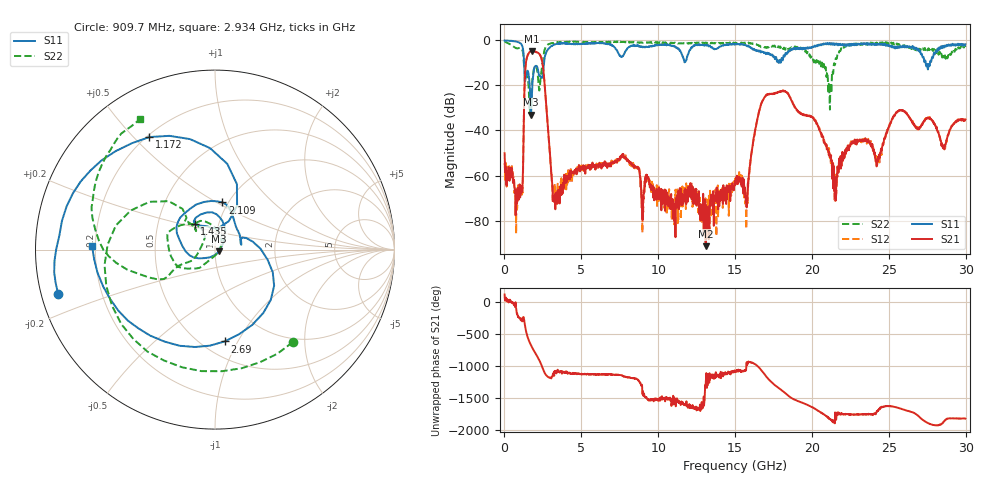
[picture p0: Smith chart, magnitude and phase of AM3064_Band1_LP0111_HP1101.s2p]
# Hz S DB R 50.0
!freq dBS11 angS11 dBS21 angS21 dBS12 angS12 dBS22 angS22
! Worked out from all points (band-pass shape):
!   1600 points, 10 MHz to 29.98 GHz, reference 50 ohm
!   highest |S21| = -4.65 dB at 1.791 GHz (marker M1); lowest = -91.4 dB at 13.09 GHz (marker M2)
!   |S21| within 3 dB of the highest: 1.46 GHz to 2.392 GHz (932.2 MHz wide, 48.4 % of centre)
!   lowest |S11| = -32.9 dB at 1.716 GHz (marker M3), VSWR 1.05, Z = 52.1 - j0.908 ohm
!   |S11| at or under -10 dB: 1.277 GHz to 2.567 GHz (1.29 GHz wide, 67.1 % of centre); 17.8465 GHz to 17.85471 GHz (8.204 MHz wide, 0.046 % of centre); 27.4 GHz to 27.68 GHz (283.1 MHz wide, 1.03 % of centre)
!   |S22| runs from -32.7 to -0.3 dB; largest |S21 - S12| = 0.009
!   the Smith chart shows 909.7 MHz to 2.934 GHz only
!   S11 on the Smith chart (normalised r, x): 909.7 MHz: 0.05, -0.14; 1.172 GHz: 0.21, +0.56; 1.435 GHz: 0.77, +0.23; 2.109 GHz: 0.94, +0.53; 2.69 GHz: 0.64, -0.88; 2.934 GHz: 0.19, +0.02
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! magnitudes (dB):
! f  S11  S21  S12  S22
! 10 MHz  0.0  -50.1  -54.5  -0.3
! 909.7 MHz  -0.8  -66.5  -63.4  -3.4
! 1.172 GHz  -2.8  -65.2  -67.7  -4.5
! 1.435 GHz  -14.8  -8.4  -8.3  -15.9
! 1.716 GHz  -32.9  -4.7  -4.7  -25.5
! 1.791 GHz  -22.5  -4.6  -4.6  -18.6
! 2.109 GHz  -11.5  -5.3  -5.3  -12.7
! 2.69 GHz  -5.8  -26.4  -26.2  -2.8
! 2.934 GHz  -3.3  -48.3  -48.2  -1.5
! 3.29 GHz  -1.8  -68.4  -66.3  -1.0
! 5.015 GHz  -1.6  -56.1  -55.5  -0.6
! 7.77 GHz  -6.2  -52.0  -51.3  -0.7
! 10 GHz  -2.1  -68.7  -71.3  -0.9
! 13.09 GHz  -2.1  -91.4  -78.4  -1.0
! 15 GHz  -1.8  -64.4  -61.3  -1.4
! 15.74 GHz  -2.2  -69.5  -83.6  -1.2
! 17.03 GHz  -5.8  -24.2  -24.3  -3.4
! 19.99 GHz  -3.3  -34.0  -34.0  -8.1
! 21.47 GHz  -1.5  -65.1  -71.9  -10.6
! 25 GHz  -2.0  -38.7  -38.1  -1.1
! 28.58 GHz  -2.9  -47.6  -47.7  -7.4
! 29.98 GHz  -1.7  -35.1  -35.4  -2.9
